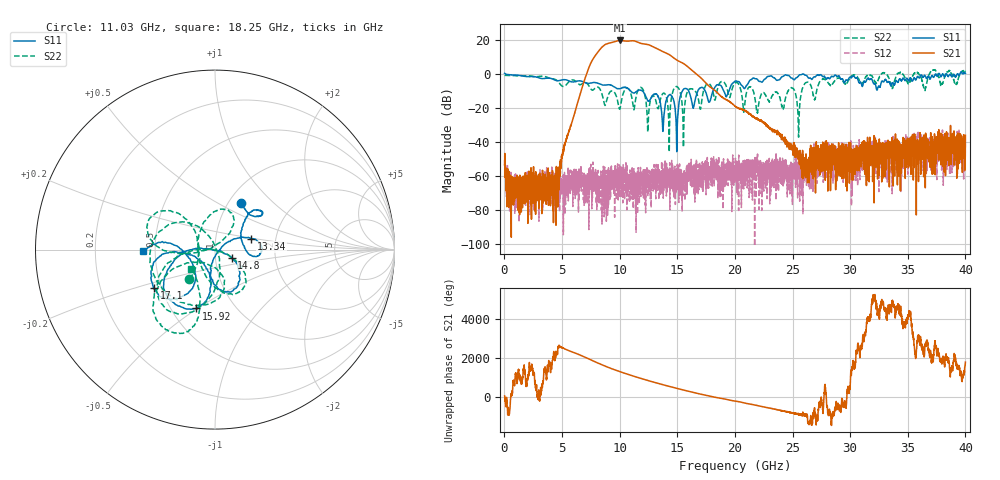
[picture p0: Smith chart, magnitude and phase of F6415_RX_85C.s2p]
!Keysight Technologies,N5245B,MY52451815,A.15.70.20
!Date: Wednesday, April 17, 2024 16:10:21
!Correction: S33(C  2-Port  )
!S43(C  2-Port  )
!S34(C  2-Port  )
!S44(C  2-Port  )
!S2P File: Measurements: S33, S43, S34, S44:
# Hz S  RI  R 50
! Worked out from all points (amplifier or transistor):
!   4000 points, 10 MHz to 40 GHz, reference 50 ohm
!   highest |S21| = 19.8 dB at 10.04 GHz (marker M1)
!   |S21| within 3 dB of that: 8.612 GHz to 12.68 GHz (4.063 GHz wide, 38.2 % of centre)
!   unconditionally stable (mu >= 1): 99.57 MHz to 25.86 GHz; 25.94 GHz to 32.7 GHz; 34.52 GHz to 35.52 GHz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
!   at 6.67 GHz: K = 1947.37, MAG = -6.1 dB, |S12| = -69.1 dB
!   at 20.01 GHz: K = 2147.98, MAG = -15.3 dB, |S12| = -61.0 dB
!   at 40 GHz: K = 151.19, MSG = 3.5 dB, |S12| = -43.1 dB
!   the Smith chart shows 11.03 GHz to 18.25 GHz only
!   S11 on the Smith chart (normalised r, x): 11.03 GHz: 1.15, +0.65; 13.34 GHz: 1.50, +0.18; 14.8 GHz: 1.20, -0.11; 15.92 GHz: 0.66, -0.49; 17.1 GHz: 0.46, -0.23; 18.25 GHz: 0.43, -0.01
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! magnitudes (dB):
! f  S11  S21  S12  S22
! 10 MHz  0.4  -53.5  -54.0  -0.7
! 1.25 GHz  -0.8  -63.5  -70.8  -1.1
! 4.42 GHz  -3.7  -70.8  -59.6  -3.2
! 6.68 GHz  -4.2  -9.2  -62.3  -6.0
! 8.18 GHz  -5.7  13.6  -62.1  -8.0
! 10.04 GHz  -8.6  19.8  -57.0  -20.0
! 11.03 GHz  -10.6  19.6  -71.1  -13.3
! 13.34 GHz  -13.5  14.6  -54.0  -20.4
! 13.76 GHz  -33.5  13.2  -68.2  -11.4
! 14.32 GHz  -12.3  11.4  -65.6  -31.8
! 14.8 GHz  -19.8  8.9  -60.7  -7.8
! 15.53 GHz  -9.0  6.2  -61.7  -43.2
! 15.92 GHz  -9.2  4.2  -58.5  -9.9
! 17.1 GHz  -7.9  -2.6  -56.1  -17.1
! 18.25 GHz  -7.9  -9.6  -52.7  -15.4
! 20.01 GHz  -4.1  -19.0  -61.0  -5.3
! 21.94 GHz  -3.1  -26.3  -58.9  -22.8
! 24.91 GHz  -2.4  -43.2  -52.7  -8.0
! 25.52 GHz  -1.1  -48.4  -51.6  -37.1
! 26.67 GHz  -3.2  -57.0  -43.5  -8.5
! 33.34 GHz  -4.4  -55.6  -44.4  -2.1
! 40 GHz  0.3  -36.1  -43.1  1.6
